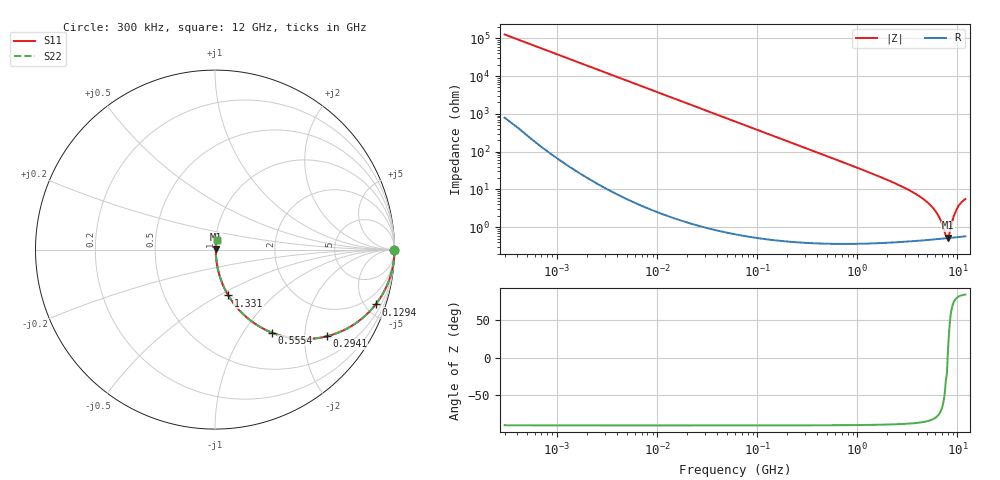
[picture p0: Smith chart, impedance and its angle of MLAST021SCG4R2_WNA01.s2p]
! MLAST021SCG4R2_WNA01  S-PARAMETER MODEL  ( General Type )
! Model Generated by TAIYO YUDEN Corporation (http://www.ty-top.com)
! Version 1.0
! TAIYO YUDEN Control No. 220901
! Copyright(c) 2022 TAIYO YUDEN CO.,LTD. All Rights Reserved.
! Product Description (link to TY-COMPAS)
! https://ds.yuden.co.jp/TYCOMPAS/or/detail?pn=MLAST021SCG4R2BWNA01&u=M
! Products Name : Multilayer Ceramic Capacitors
! Characteristics :
!  Capacitance : 4.2 pF , Rated Voltage : 25V , TCC : CG / C0G
!  Case Size : 0.25 x 0.125 / 0.0098 x 0.0049 [mm/inch] , Thickness : 0.125 / 0.0049 [mm/inch]
!  (Conditions: Temperature = 25 degC , DC Bias Current/Voltage = 0A / 0V)
! External Node Assignments :
!  1  o---| |---o  2
! GND o---------o GND
! Frequency Range : 0.3MHz  -  12000MHz  [ 401 STEP ]
# MHz S RI R 50
! Freq[MHz].  S11 Real  S11 Imag  S21 Real  S21 Imag  S12 Real  S12 Imag  S22 Real  S22 Imag
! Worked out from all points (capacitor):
!   401 points, 300 kHz to 12 GHz, reference 50 ohm
!   read as one part in series: C = 4.2 pF near 316.3 kHz
!   lowest |Z| = 527 mohm at 8.065 GHz (marker M1)
!   series resonance near 7.982 GHz, so ESL is about 95 pH
!   S11 on the Smith chart (normalised r, x): 300 kHz: open; 129.4 MHz: 1.01, -5.86; 294.1 MHz: 1.01, -2.57; 555.4 MHz: 1.01, -1.36; 1.331 GHz: 1.01, -0.55; 12 GHz: 1.01, +0.11
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0.3  1 -0.000792  5.58e-06 0.000792  5.58e-06 0.000792  1 -0.000792
1.769972  1 -0.00467  2.72e-05 0.00467  2.72e-05 0.00467  1 -0.00467
10.44266  0.9992 -0.0275  0.000777 0.0275  0.000777 0.0275  0.9992 -0.0275
60  0.9754 -0.1544  0.0246 0.1544  0.0246 0.1544  0.9754 -0.1544
129.3602  0.8952 -0.3055  0.1048 0.3055  0.1048 0.3055  0.8952 -0.3055
192.4766  0.7942 -0.4032  0.2058 0.4032  0.2058 0.4032  0.7942 -0.4032
294.0765  0.6231 -0.4831  0.3769 0.4831  0.3769 0.4831  0.6231 -0.4831
353.9943  0.5329 -0.4972  0.4671 0.4972  0.4671 0.4972  0.5329 -0.4972
555.3718  0.3164 -0.4624  0.6836 0.4624  0.6836 0.4624  0.3164 -0.4624
848.5281  0.1651 -0.3672  0.8349 0.3672  0.8349 0.3672  0.1651 -0.3672
1331.232  0.074 -0.2552  0.926 0.2552  0.926 0.2552  0.074 -0.2552
2088.533  0.0312 -0.1628  0.9688 0.1628  0.9688 0.1628  0.0312 -0.1628
3642.919  0.0108 -0.0806  0.9892 0.0806  0.9892 0.0806  0.0108 -0.0806
5140.631  0.00634 -0.042  0.9937 0.042  0.9937 0.042  0.00634 -0.042
6188.031  0.00532 -0.0234  0.9947 0.0234  0.9947 0.0234  0.00532 -0.0234
6699.894  0.00511 -0.0157  0.9949 0.0157  0.9949 0.0157  0.00511 -0.0157
7648.807  0.00504 -0.00301  0.995 0.00301  0.995 0.00301  0.00504 -0.00301
8064.993  0.0051 0.0012  0.9949 -0.0012  0.9949 -0.0012  0.0051 0.0012
8281.503  0.00515 0.00388  0.9948 -0.00388  0.9948 -0.00388  0.00515 0.00388
9708.23  0.00606 0.0266  0.9939 -0.0266  0.9939 -0.0266  0.00606 0.0266
10793.46  0.00733 0.0426  0.9927 -0.0426  0.9927 -0.0426  0.00733 0.0426
12000  0.00866 0.0544  0.9913 -0.0544  0.9913 -0.0544  0.00866 0.0544
